(* Logix 5000 AddOnInstructionDefinition export; software revision 16.04; part 2 of 2 *)
(* tags used below, declared in another part *)
   Velocity : DINT;   // Velocity
   OS_LoadStart : BOOL;
(* AKD_Set_Velocity, continued *)

ROUTINE Prescan   (* ladder *)
// Prescan
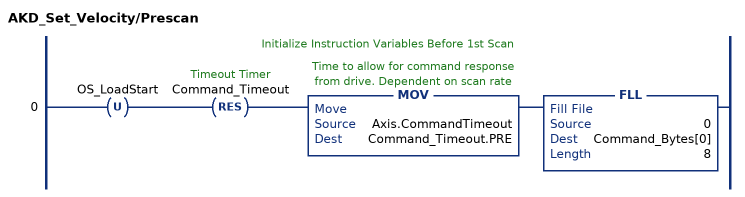
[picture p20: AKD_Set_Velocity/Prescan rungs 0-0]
   // Initialize Instruction Variables Before 1st Scan
   0: OTU(OS_LoadStart)RES(Command_Timeout)MOV(Axis.CommandTimeout,Command_Timeout.PRE)FLL(0,Command_Bytes[0],8);
END_ROUTINE
END_ADD_ON_INSTRUCTION

ADD_ON_INSTRUCTION AKD_Jog   (* revision 2.3, ExecutePrescan, ExecuteEnableInFalse *)
// Motion Axis Jog
// Revision note:
// Remove unused IP output
VAR_IN_OUT
   Axis : AKD_Axis; {required}
END_VAR
VAR_INPUT
   Accel : DINT; {required}   // Acceleration
   Decel : DINT; {required}   // Deceleration
   Direction : BOOL; {required}   // 1=Forward/Positive, 0=Reverse/Negative
   Speed : DINT; {required}   // Jog Speed
END_VAR
VAR_OUTPUT
   DN : BOOL; {visible}   // Command Successfully Initiated
   ER : BOOL; {visible}   // Error
END_VAR
VAR
   Accel_Internal : DINT;   // Scaled Accel Value for Drive
   Set_Enable : AKD_Enable;
   Set_Accel : AKD_Set_Accel;
   Set_Decel : AKD_Set_Decel;
   Set_Velocity : AKD_Set_Velocity;
   Step : SINT;   // Sequence Step Number
   Command_Axis_Number : SINT;
   Response_Axis_Number : SINT;
   OS_Start_Sequence : BOOL;
   Command_Bytes : SINT[64];
   ErrorData : SINT[8];
   Command_Timeout : TIMER;
END_VAR

ROUTINE EnableInFalse   (* ladder *)
// EnableIn_False
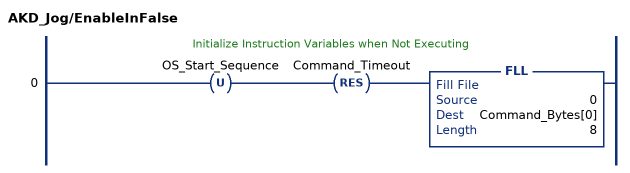
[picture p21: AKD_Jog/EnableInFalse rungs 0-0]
   // Initialize Instruction Variables when Not Executing
   0: OTU(OS_Start_Sequence)RES(Command_Timeout)FLL(0,Command_Bytes[0],8);
END_ROUTINE

ROUTINE Logic   (* ladder *)
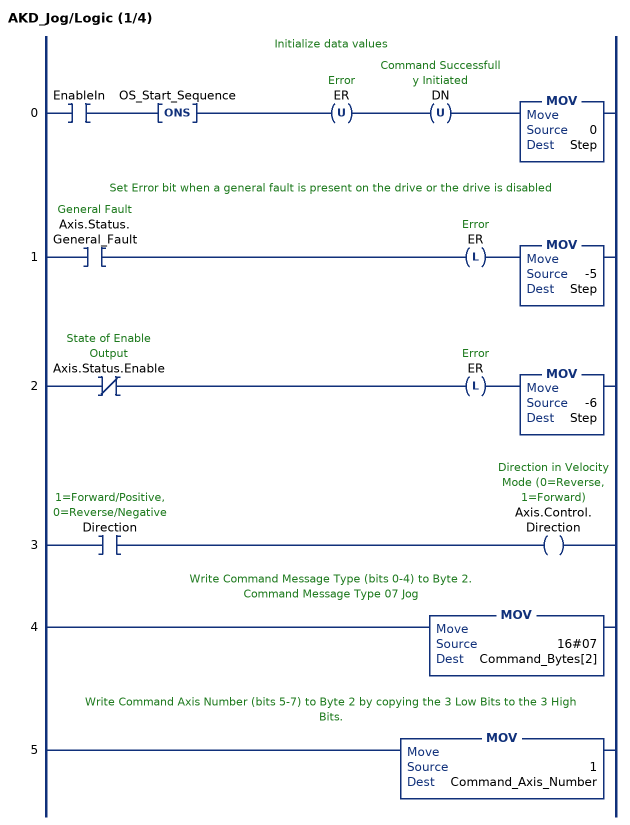
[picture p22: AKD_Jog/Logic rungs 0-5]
   // Initialize data values
   0: XIC(EnableIn)ONS(OS_Start_Sequence)OTU(ER)OTU(DN)MOV(0,Step);
   // Set Error bit when a general fault is present on the drive or the drive is disabled
   1: XIC(Axis.Status.General_Fault)OTL(ER)MOV(-5,Step);
   2: XIO(Axis.Status.Enable)OTL(ER)MOV(-6,Step);
   3: XIC(Direction)OTE(Axis.Control.Direction);
   // Write Command Message Type (bits 0-4) to Byte 2.
   // Command Message Type 07 Jog
   4: MOV(16#07,Command_Bytes[2]);
   // Write Command Axis Number (bits 5-7) to Byte 2 by copying the 3 Low Bits to the 3 High Bits.
   5: MOV(1,Command_Axis_Number);
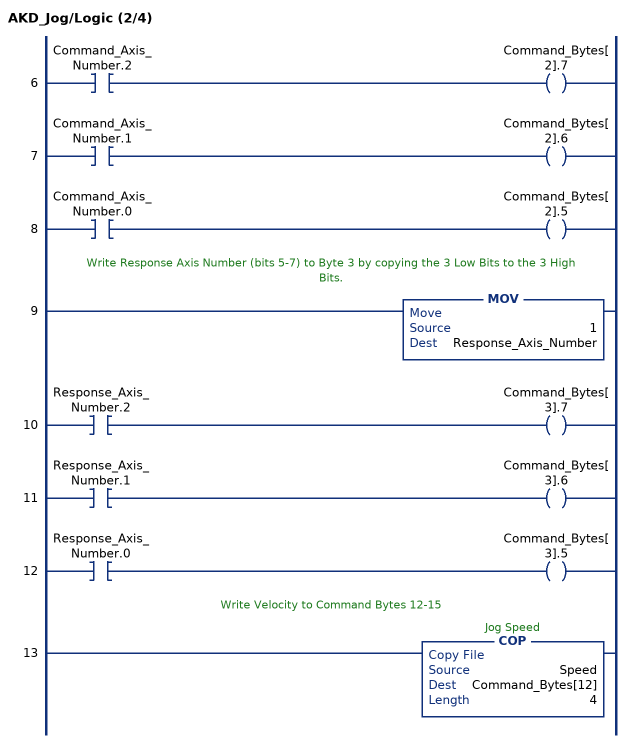
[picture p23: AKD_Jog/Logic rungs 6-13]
   6: XIC(Command_Axis_Number.2)OTE(Command_Bytes[2].7);
   7: XIC(Command_Axis_Number.1)OTE(Command_Bytes[2].6);
   8: XIC(Command_Axis_Number.0)OTE(Command_Bytes[2].5);
   // Write Response Axis Number (bits 5-7) to Byte 3 by copying the 3 Low Bits to the 3 High Bits.
   9: MOV(1,Response_Axis_Number);
   10: XIC(Response_Axis_Number.2)OTE(Command_Bytes[3].7);
   11: XIC(Response_Axis_Number.1)OTE(Command_Bytes[3].6);
   12: XIC(Response_Axis_Number.0)OTE(Command_Bytes[3].5);
   // Write Velocity to Command Bytes 12-15
   13: COP(Speed,Command_Bytes[12],4);
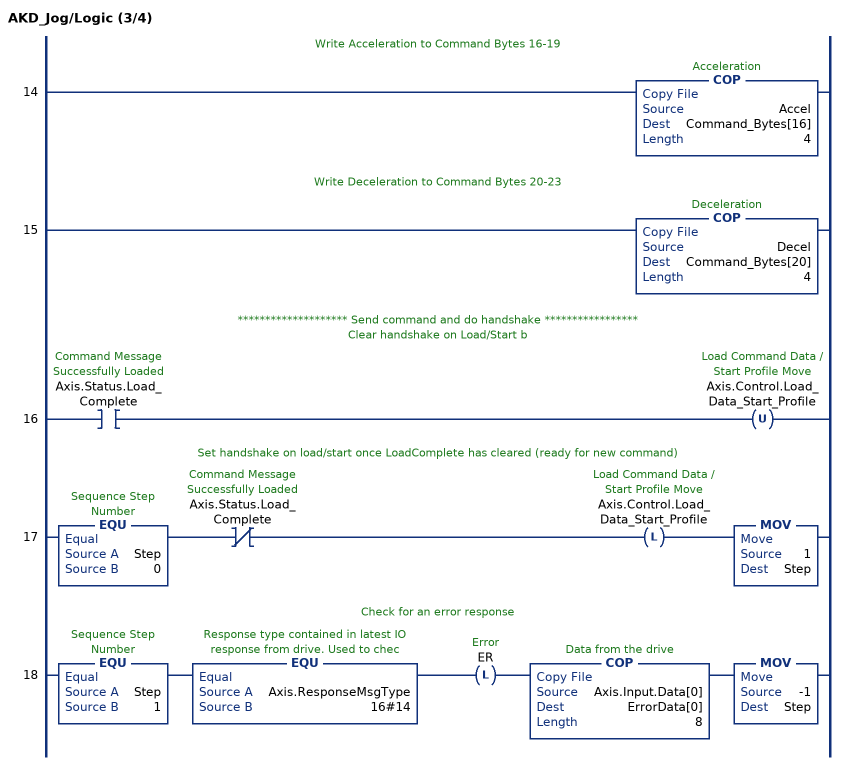
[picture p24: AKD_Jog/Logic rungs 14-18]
   // Write Acceleration to Command Bytes 16-19
   14: COP(Accel,Command_Bytes[16],4);
   // Write Deceleration to Command Bytes 20-23
   15: COP(Decel,Command_Bytes[20],4);
   // ******************** Send command and do handshake *****************
   // Clear handshake on Load/Start b
   16: XIC(Axis.Status.Load_Complete)OTU(Axis.Control.Load_Data_Start_Profile);
   // Set handshake on load/start once LoadComplete has cleared (ready for new command)
   17: EQU(Step,0)XIO(Axis.Status.Load_Complete)OTL(Axis.Control.Load_Data_Start_Profile)MOV(1,Step);
   // Check for an error response
   18: EQU(Step,1)EQU(Axis.ResponseMsgType,16#14)OTL(ER)COP(Axis.Input.Data[0],ErrorData[0],8)MOV(-1,Step);
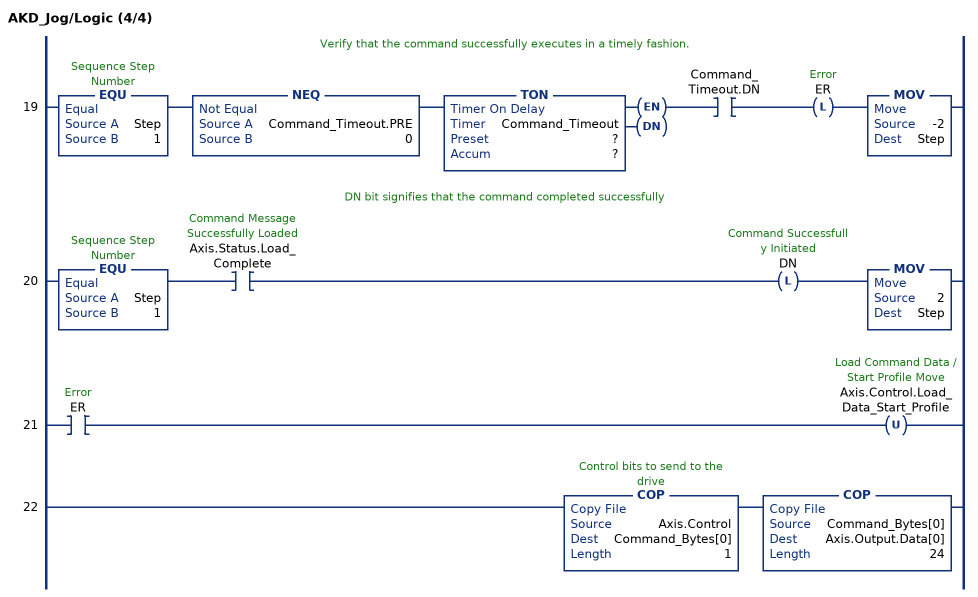
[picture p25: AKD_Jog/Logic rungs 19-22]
   // Verify that the command successfully executes in a timely fashion.
   19: EQU(Step,1)NEQ(Command_Timeout.PRE,0)TON(Command_Timeout,?,?)XIC(Command_Timeout.DN)OTL(ER)MOV(-2,Step);
   // DN bit signifies that the command completed successfully
   20: EQU(Step,1)XIC(Axis.Status.Load_Complete)OTL(DN)MOV(2,Step);
   21: XIC(ER)OTU(Axis.Control.Load_Data_Start_Profile);
   22: COP(Axis.Control,Command_Bytes[0],1)COP(Command_Bytes[0],Axis.Output.Data[0],24);
END_ROUTINE

ROUTINE Prescan   (* ladder *)
// Prescan
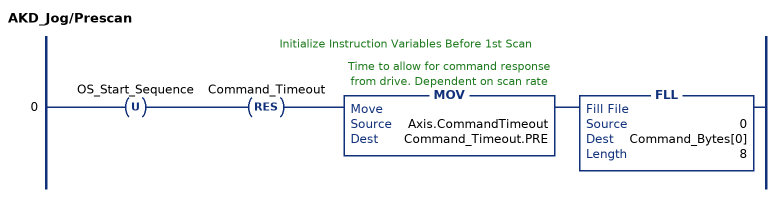
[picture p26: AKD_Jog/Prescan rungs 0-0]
   // Initialize Instruction Variables Before 1st Scan
   0: OTU(OS_Start_Sequence)RES(Command_Timeout)MOV(Axis.CommandTimeout,Command_Timeout.PRE)FLL(0,Command_Bytes[0],8);
END_ROUTINE
END_ADD_ON_INSTRUCTION
